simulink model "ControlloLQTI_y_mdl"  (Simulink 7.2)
settings: Solver=ode45  StartTime=0.0  StopTime=10.0  RelTol=1e-3
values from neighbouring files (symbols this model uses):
  A = [0 1; -2 1]    [RegolazioneOttimaTempoInfinita_Integrale.m]    (also in RegolazioneOttimaTempoInfinita_TempoDiscreto.m; RegolazioneOttimaTempoInfinita_uscita.m; RegolazioneOttimaTempoInfinita_uscita_osservatore.m; RegolazioneOttimaTempoInfinita.m)
  B = [0; 1]    [RegolazioneOttimaTempoInfinita_Integrale.m]    (also in RegolazioneOttimaTempoInfinita_TempoDiscreto.m; RegolazioneOttimaTempoInfinita_uscita.m; RegolazioneOttimaTempoInfinita_uscita_osservatore.m; RegolazioneOttimaTempoInfinita.m)
  C = [1 0]    [RegolazioneOttimaTempoInfinita_Integrale.m]    (also in RegolazioneOttimaTempoInfinita_TempoDiscreto.m; RegolazioneOttimaTempoInfinita_uscita.m = [0 1]; RegolazioneOttimaTempoInfinita_uscita_osservatore.m = [0 1]; RegolazioneOttimaTempoInfinita.m)
  Kyu = -inv(C*inv(A-B*K)*B)    [ControlloOttimoTempoInfinito.m]    (also in ControlloOttimoTempoInfinito_TempoDiscreto.m)
  X0 = [2;-3]    [RegolazioneOttimaTempoInfinita_Integrale.m]    (also in RegolazioneOttimaTempoInfinita_TempoDiscreto.m; RegolazioneOttimaTempoInfinita_uscita.m; RegolazioneOttimaTempoInfinita_uscita_osservatore.m; RegolazioneOttimaTempoInfinita.m)
  yp = 4    [ControlloOttimoTempoInfinito.m]    (also in ControlloOttimoTempoInfinito_TempoDiscreto.m)
undefined symbols (not defined in the file or in its folder): K

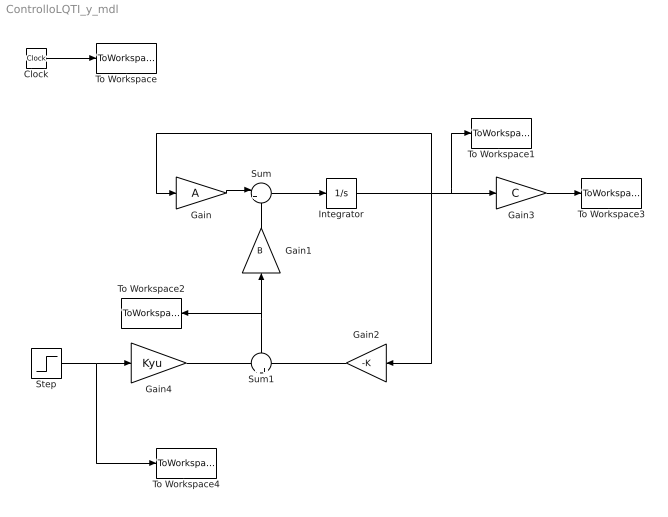
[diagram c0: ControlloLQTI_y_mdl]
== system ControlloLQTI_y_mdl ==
  Clock : Clock
  Gain : Gain  Gain=A  Multiplication=Matrix(K*u)  ParameterDataType=sfix(16)  ParameterScaling=2^0  OutDataType=sfix(16)  OutScaling=2^0
  Gain1 : Gain  Orientation=up  Gain=B  Multiplication=Matrix(K*u)  ParameterDataType=sfix(16)  ParameterScaling=2^0  OutDataType=sfix(16)  OutScaling=2^0
  Gain2 : Gain  Orientation=left  Gain=-K  Multiplication=Matrix(K*u)  ParameterDataType=sfix(16)  ParameterScaling=2^0  OutDataType=sfix(16)  OutScaling=2^0
  Gain3 : Gain  Gain=C  Multiplication=Matrix(K*u)  ParameterDataType=sfix(16)  ParameterScaling=2^0  OutDataType=sfix(16)  OutScaling=2^0
  Gain4 : Gain  Gain=Kyu  Multiplication=Matrix(K*u)  ParameterDataType=sfix(16)  ParameterScaling=2^0  OutDataType=sfix(16)  OutScaling=2^0
  Integrator : Integrator  InitialCondition=X0
  Step : Step  Time=5  After=yp  SampleTime=0
  Sum : Sum  Inputs=|++  OutDataType=sfix(16)  OutScaling=2^0
  Sum1 : Sum  Orientation=up  OutDataType=sfix(16)  OutScaling=2^0
  To Workspace : ToWorkspace  VariableName=time  SampleTime=-1  SaveFormat=Array
  To Workspace1 : ToWorkspace  VariableName=X  SampleTime=-1  SaveFormat=Array
  To Workspace2 : ToWorkspace  VariableName=u  SampleTime=-1  SaveFormat=Array
  To Workspace3 : ToWorkspace  VariableName=y  SampleTime=-1  SaveFormat=Array
  To Workspace4 : ToWorkspace  VariableName=yd  SampleTime=-1  SaveFormat=Array
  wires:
  Gain/1 -> Sum/1
  Integrator/1 -> Gain/1, Gain2/1, To Workspace1/1, Gain3/1
  Gain1/1 -> Sum/2
  Sum/1 -> Integrator/1
  Clock/1 -> To Workspace/1
  Gain3/1 -> To Workspace3/1
  Sum1/1 -> Gain1/1, To Workspace2/1
  Gain2/1 -> Sum1/2
  Gain4/1 -> Sum1/1
  Step/1 -> Gain4/1, To Workspace4/1
